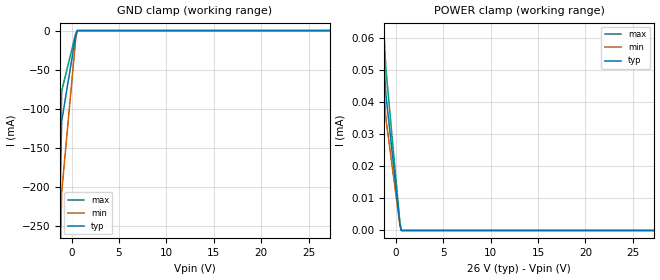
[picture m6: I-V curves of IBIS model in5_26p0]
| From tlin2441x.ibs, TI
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|   in5_26p0 Model
[Model]   in5_26p0
Model_type   Input
Vinl = 23
Vinh = 24
|   typ   min   max
C_comp   4.302pF   4.223pF   4.302pF
|  Where Nom  PVT is Nominal Process, 26.0V,   27C
|   Fast PVT is Strong Process,  28.0,   -40C
|   Slow PVT is Weak Process,   24.0V,   150C
[Model spec]
|subparameter
Vinl   23   21   25
Vinh   24   22   26
[Voltage Range]   26   24   28
|Junction Temperature
[Temperature Range]   27   150   -40
[Power Clamp Reference]   26   24   28
[GND Clamp Reference]   0   0   0
[GND Clamp]
|   Voltage   I(typ)   I(min)   I(max)
-26V      -19.76A    -19.5A     -19.96A
-2.132V   -769.3mA   -884mA     -726.3mA
-1.04V    -115.9mA   -206.8mA   -77.31mA
442mV     -5.799mA   -10.34mA   -3.869mA
598mV     -3.222uA   -2.673uA   -4.387uA
52V       0A         0A         0A
[POWER Clamp]
|   Voltage   I(typ)   I(min)   I(max)
-26V      1.276mA    1.143mA    1.464mA
-2.132V   95.13uA    81.16uA    111uA
-1.04V    42.4uA     34.94uA    50.4uA
442mV     2uA        1.635uA    2.391uA
598mV     0A         0A         0A
52V       0A         0A         0A
